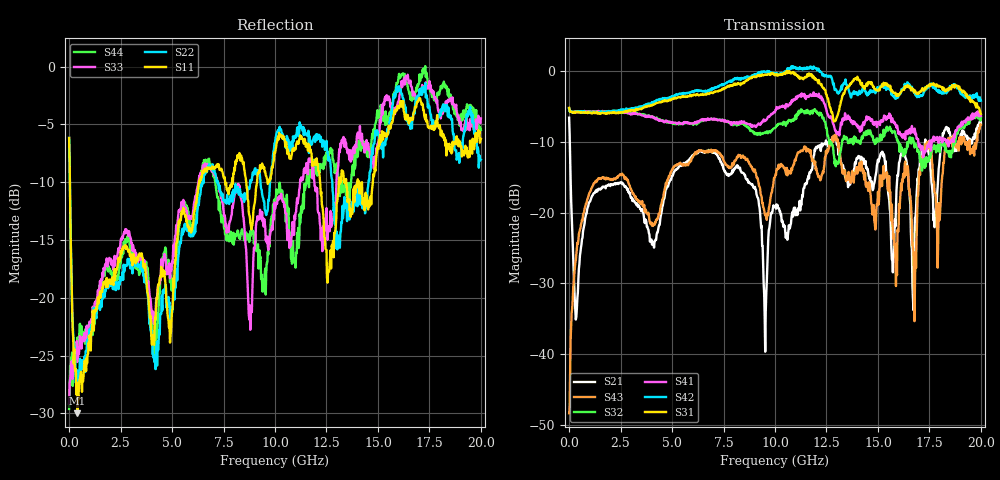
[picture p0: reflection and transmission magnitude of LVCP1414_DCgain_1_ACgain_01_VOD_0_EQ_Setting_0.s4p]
!Agilent Technologies,N5230A,MY46400459,A.07.50.48
!Agilent N5230A: A.07.50.48
!Date: Tuesday, April 17, 2012 18:45:02
!Correction: S11(Full 4 Port(1,2,3,4))
!S12(Full 4 Port(1,2,3,4))
!S13(Full 4 Port(1,2,3,4))
!S14(Full 4 Port(1,2,3,4))
!S21(Full 4 Port(1,2,3,4))
!S22(Full 4 Port(1,2,3,4))
!S23(Full 4 Port(1,2,3,4))
!S24(Full 4 Port(1,2,3,4))
!S31(Full 4 Port(1,2,3,4))
!S32(Full 4 Port(1,2,3,4))
!S33(Full 4 Port(1,2,3,4))
!S34(Full 4 Port(1,2,3,4))
!S41(Full 4 Port(1,2,3,4))
!S42(Full 4 Port(1,2,3,4))
!S43(Full 4 Port(1,2,3,4))
!S44(Full 4 Port(1,2,3,4))
!S4P File: Measurements: <S11,S12,S13,S14>,
!<S21,S22,S23,S24>,
!<S31,S32,S33,S34>,
!<S41,S42,S43,S44>:
# Hz S  dB  R 50
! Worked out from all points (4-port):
!   801 points, 300 kHz to 20 GHz, reference 50 ohm
!   strongest paths, dB at 300 kHz, 5 GHz, 10 GHz, 15 GHz, 20 GHz:
!     S31: -5.2, -3.9, -0.5, -2.7, -6.0
!     S42: -5.3, -3.5, -0.3, -2.3, -4.2
!     S41: -5.2, -7.2, -5.7, -7.2, -6.3
!     S32: -5.3, -7.3, -8.0, -9.9, -6.6
!     S43: -48.4, -13.9, -14.9, -17.0, -7.5
!     S21: -6.5, -14.8, -19.2, -12.5, -7.3
!   lowest |S11| = -30.0 dB at 400.3 MHz (marker M1), VSWR 1.07, Z = 52.9 + j1.49 ohm
!   |S11| at or under -10 dB: 37.68 MHz to 6.313 GHz (6.275 GHz wide, 198 % of centre); 8.603 GHz to 9.127 GHz (524.7 MHz wide, 5.92 % of centre); 12.19 GHz to 13.1 GHz (910.4 MHz wide, 7.2 % of centre)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
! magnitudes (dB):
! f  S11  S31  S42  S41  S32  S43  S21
! 300 kHz  -6.2  -5.2  -5.3  -5.2  -5.3  -48.4  -6.5
! 400.3 MHz  -30.0  -5.7  -5.7  -5.7  -5.7  -24.2  -32.1
! 10.03 GHz  -7.2  -0.5  -0.3  -5.4  -7.9  -14.5  -19.0
! 12.88 GHz  -14.4  -7.1  -2.2  -7.8  -12.1  -9.2  -9.4
! 14.03 GHz  -9.7  -1.0  -3.3  -8.0  -10.0  -13.5  -12.3
! 16.78 GHz  -3.8  -2.6  -3.1  -8.1  -10.8  -35.3  -23.6
! 20 GHz  -6.3  -6.0  -4.2  -6.3  -6.6  -7.5  -7.3
